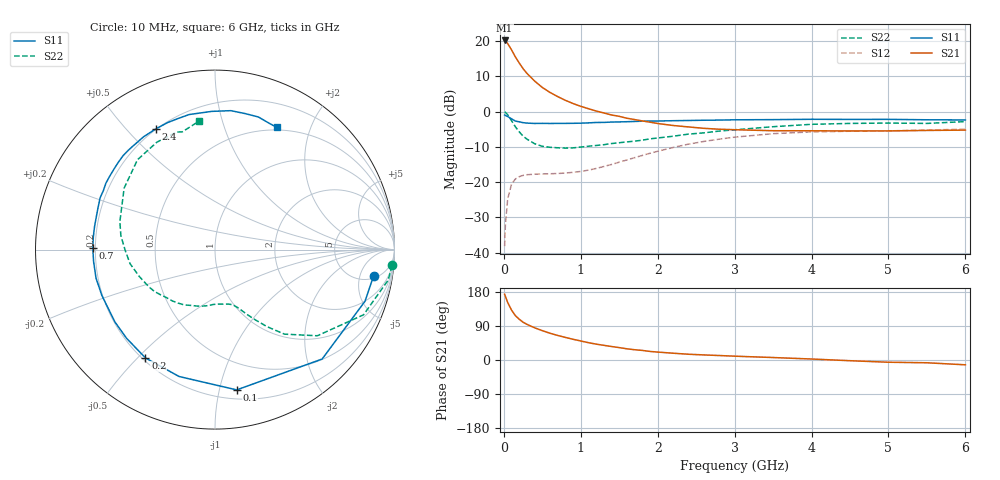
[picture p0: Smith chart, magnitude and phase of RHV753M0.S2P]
! SIEMENS Small Signal Semiconductors
! BFR106
! Si NPN RF Bipolar Junction Transistor in SOT23
! VCE = 0.75 V  IC = 3 mA
! Common Emitter S-Parameters:  August  1996
# GHz  S  MA  R  50
!  f  S11  S21  S12  S22
! GHz  MAG  ANG  MAG  ANG  MAG  ANG  MAG  ANG
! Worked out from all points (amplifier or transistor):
!   36 points, 10 MHz to 6 GHz, reference 50 ohm
!   highest |S21| = 20.2 dB at 10 MHz (marker M1)
!   |S21| within 3 dB of that: start of sweep to 108.3 MHz
!   unconditionally stable (mu >= 1): 682.1 MHz to end of sweep
!   at 250 MHz: K = 0.41, MSG = 15.2 dB, |S12| = -18.1 dB
!   at 1.4 GHz: K = 1.28, MAG = 3.8 dB, |S12| = -15.0 dB
!   at 6 GHz: K = 1.03, MAG = -1.2 dB, |S12| = -5.0 dB
!   S11 on the Smith chart (normalised r, x): 10 MHz: 6, -8; 100 MHz: 0.27, -1.13; 200 MHz: 0.21, -0.53; 700 MHz: 0.19, +0.01; 2.4 GHz: 0.20, +0.60; 6 GHz: 0.47, +1.52
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0.01  0.8955 -9.5  10.26 173.5  0.0123 86.5  0.9919 -5.1
0.02  0.8839 -19.0  10.15 168.4  0.0247 81.6  0.9788 -10.1
0.05  0.8532 -45.6  9.27 151.7  0.0575 65.6  0.9039 -23.7
0.1  0.7909 -81.2  7.542 131.8  0.0931 48.9  0.7453 -40.1
0.15  0.7348 -105.8  5.991 117.0  0.1107 37.8  0.6096 -50.6
0.2  0.7172 -122.7  4.911 107.6  0.1194 31.7  0.5175 -56.0
0.25  0.6978 -134.9  4.082 99.7  0.1245 27.8  0.4491 -60.3
0.3  0.6881 -144.1  3.498 94.1  0.1272 25.9  0.407 -63.4
0.4  0.6801 -157.9  2.721 85.0  0.1294 23.6  0.3505 -68.2
0.5  0.6817 -166.5  2.205 77.4  0.1305 23.3  0.3223 -72.2
0.6  0.6798 -174.4  1.875 70.6  0.1312 24.3  0.3116 -76.7
0.7  0.6809 179.2  1.636 64.8  0.1324 26.5  0.3069 -82.0
0.9  0.6832 169.2  1.304 54.7  0.1376 32.2  0.3059 -92.0
1.1  0.6928 160.0  1.101 45.7  0.1478 38.5  0.323 -102.8
1.6  0.7197 141.5  0.806 29.5  0.2062 49.0  0.3722 -129.9
2.2  0.7439 122.3  0.636 17.9  0.3099 46.7  0.4478 -160.5
2.4  0.749 116.2  0.607 15.2  0.3455 43.8  0.4797 -170.6
2.8  0.7589 105.6  0.563 11.8  0.4071 36.6  0.5298 171.7
3.5  0.7703 91.3  0.536 6.5  0.4868 23.0  0.6113 145.9
4.5  0.7762 77.3  0.532 -1.9  0.5273 6.2  0.6805 118.4
5.5  0.7666 67.2  0.541 -7.3  0.5485 -3.2  0.6808 105.5
6  0.7628 63.3  0.547 -12.7  0.5635 -9.8  0.7224 96.9
